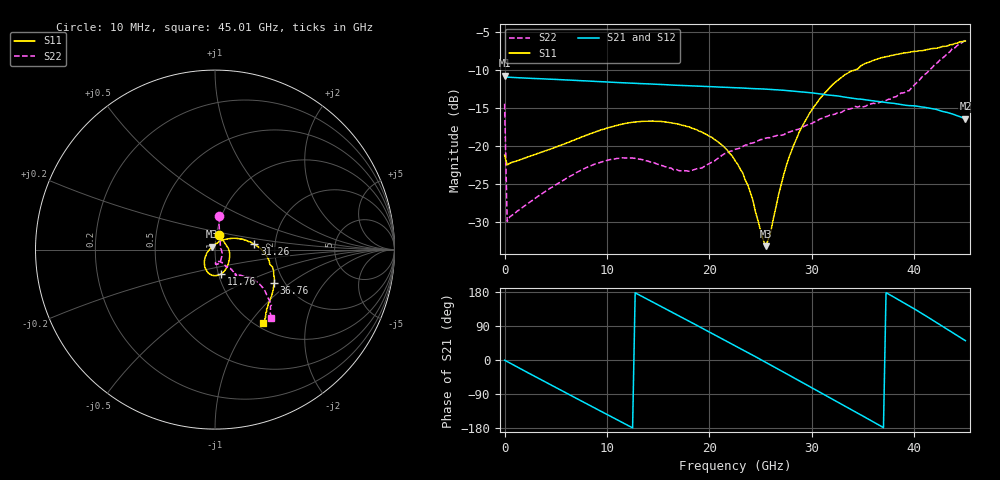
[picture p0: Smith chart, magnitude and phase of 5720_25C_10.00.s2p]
! Device:  ADRF5720
! Description: 0.5dB LSB GaAs MMIC 6-bit Digital Attenuator
! Frequency:  0.000009 -  40 GHz
! Ports:
!	RF1	= Port 1
!	RF2	= Port 2
! Vdd:  3.3 Volt
! Vss:  -3.3 Volt
! Control:  0/3.3 Volt
! State:  10.00 dB attenuation
! Data:  The device was measured using G-S-G Probes on a matrix board.
!  Data was collected using an calibrated 4 port network analyzer.
!  The reference plane for this measurement is at the launchers.
! Note:  Analog Devices supplies this data as a sample of measured data
!  for this product.  Your particular data for this product may vary.
!  Data was taken at 25 degrees C.
!  Analog Devices reserves the right to change this data at anytime.
# GHZ S DB R 45.0
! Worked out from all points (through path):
!   181 points, 10 MHz to 45.01 GHz, reference 45 ohm
!   highest |S21| = -10.78 dB at 10 MHz (marker M1); lowest = -16.4 dB at 45.01 GHz (marker M2)
!   group delay of S21, straight-line fit = 40.8 ps
!   lowest |S11| = -33.2 dB at 25.51 GHz (marker M3), VSWR 1.04, Z = 43.7 + j1.39 ohm
!   |S11| at or under -10 dB: start of sweep to 34.26 GHz
!   |S22| runs from -30.0 to -6.1 dB; largest |S21 - S12| = 0.00033
!   S11 on the Smith chart (normalised r, x): 10 MHz: 1.03, +0.17; 11.76 GHz: 1.03, -0.29; 31.26 GHz: 1.56, +0.10; 36.76 GHz: 1.77, -0.77; 45.01 GHz: 1.08, -1.17
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0.01  -21.23 74.5  -10.78 -0.5  -10.78 -0.5  -14.47 84.0
0.26  -22.53 4.8  -10.96 -4.0  -10.97 -4.0  -29.96 12.9
4.26  -20.54 -31.0  -11.22 -61.9  -11.22 -61.9  -25.77 -41.9
7.76  -18.73 -53.6  -11.44 -111.8  -11.44 -111.8  -23.02 -64.8
11.76  -17.07 -76.3  -11.72 -168.5  -11.72 -168.5  -21.60 -82.8
15.26  -16.79 -94.4  -11.92 141.7  -11.93 141.7  -22.55 -88.3
19.01  -18.08 -112.9  -12.15 88.2  -12.15 88.2  -22.95 -69.5
21.26  -19.92 -125.7  -12.28 55.8  -12.29 55.9  -21.24 -61.1
22.76  -22.42 -138.8  -12.37 34.1  -12.37 34.2  -20.41 -58.4
24.01  -26.14 -156.6  -12.45 15.9  -12.45 16.0  -19.68 -57.9
25.51  -33.22 133.3  -12.54 -6.1  -12.54 -6.0  -18.99 -57.5
26.01  -31.28 94.0  -12.58 -13.4  -12.58 -13.4  -18.94 -56.4
26.76  -26.48 64.2  -12.64 -24.6  -12.64 -24.6  -18.57 -54.6
27.76  -21.62 44.4  -12.75 -39.5  -12.75 -39.5  -18.21 -53.2
30.26  -14.78 16.3  -13.07 -77.0  -13.08 -77.0  -16.86 -50.5
31.26  -13.08 7.7  -13.25 -92.0  -13.26 -92.0  -16.22 -50.3
34.01  -10.11 -13.6  -13.75 -133.2  -13.75 -133.1  -15.02 -49.3
36.76  -8.42 -29.5  -14.20 -174.6  -14.21 -174.6  -14.21 -47.9
37.76  -8.11 -34.3  -14.38 170.2  -14.38 170.3  -13.84 -44.6
39.51  -7.69 -41.5  -14.71 143.1  -14.71 143.2  -12.75 -40.9
41.76  -7.20 -48.1  -15.10 106.2  -15.11 106.2  -9.71 -38.2
45.01  -6.19 -56.6  -16.43 51.1  -16.43 51.1  -6.13 -50.5
